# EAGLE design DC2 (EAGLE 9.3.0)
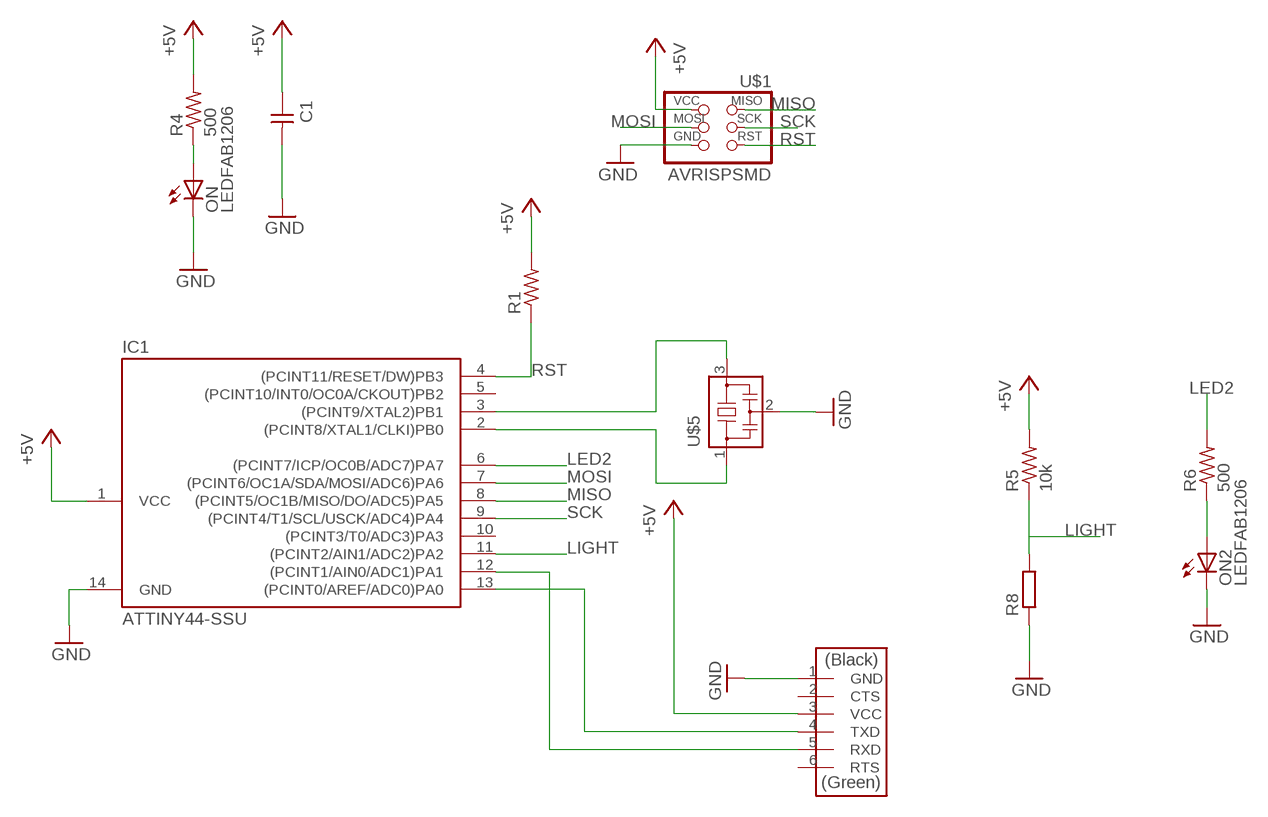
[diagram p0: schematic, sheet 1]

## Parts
C1  CAP-UNPOLARIZEDFAB  [C1206FAB]
IC1  ATTINY44-SSU  [SOIC14]
ON  LEDFAB1206  [LED1206FAB]
ON2  LEDFAB1206  [LED1206FAB]
R1  RES-US1206FAB  [R1206FAB]
R4  500  RES-US1206FAB  [R1206FAB]
R5  10k  RES-US1206FAB  [R1206FAB]
R6  500  RES-US1206FAB  [R1206FAB]
R8  R-EU_0207/10  [0207/10]
U$1  AVRISPSMD  [2X03SMD]
U$2  FTDI-SMD-HEADER  [1X06SMD]
U$5  RESONATOR  [EFOBM]

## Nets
+5V: C1.1 IC1.1(VCC) R1.2 R4.2 R5.2 U$1.2(VCC) U$2.3(VCC)
GND: C1.2 IC1.14(GND) ON2.2(C) ON.2(C) R8.1 U$1.6(GND) U$2.1(GND) U$5.2
LED2: IC1.6((PCINT7/ICP/OC0B/ADC7)PA7) R6.2
LIGHT: IC1.11((PCINT2/AIN1/ADC2)PA2) R5.1 R8.2
MISO: IC1.8((PCINT5/OC1B/MISO/DO/ADC5)PA5) U$1.1(MISO)
MOSI: IC1.7((PCINT6/OC1A/SDA/MOSI/ADC6)PA6) U$1.4(MOSI)
N$1: IC1.2((PCINT8/XTAL1/CLKI)PB0) U$5.1
N$3: IC1.13((PCINT0/AREF/ADC0)PA0) U$2.4(TXD)
N$4: IC1.12((PCINT1/AIN0/ADC1)PA1) U$2.5(RXD)
N$5: IC1.3((PCINT9/XTAL2)PB1) U$5.3
N$6: ON2.1(A) R6.1
N$9: ON.1(A) R4.1
RST: IC1.4((PCINT11/RESET/DW)PB3) R1.1 U$1.5(RST)
SCK: IC1.9((PCINT4/T1/SCL/USCK/ADC4)PA4) U$1.3(SCK)
Unconnected: IC1.5((PCINT10/INT0/OC0A/CKOUT)PB2) IC1.10((PCINT3/T0/ADC3)PA3) U$2.2(CTS) U$2.6(RTS)

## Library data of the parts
C1 = fab:CAP-UNPOLARIZED
IC1 = fab:ATTINY44
ON ON2 = fab:LED: LED
R1 R4-R6 = fab:RES-US: Resistor (US Symbol)
R8 = rcl:R-EU_: RESISTOR, European symbol; SPICEPREFIX: R
U$1 = fab:AVRISP
U$2 = fab:FTDI-SMD-HEADER
U$5 = fab:RESONATOR

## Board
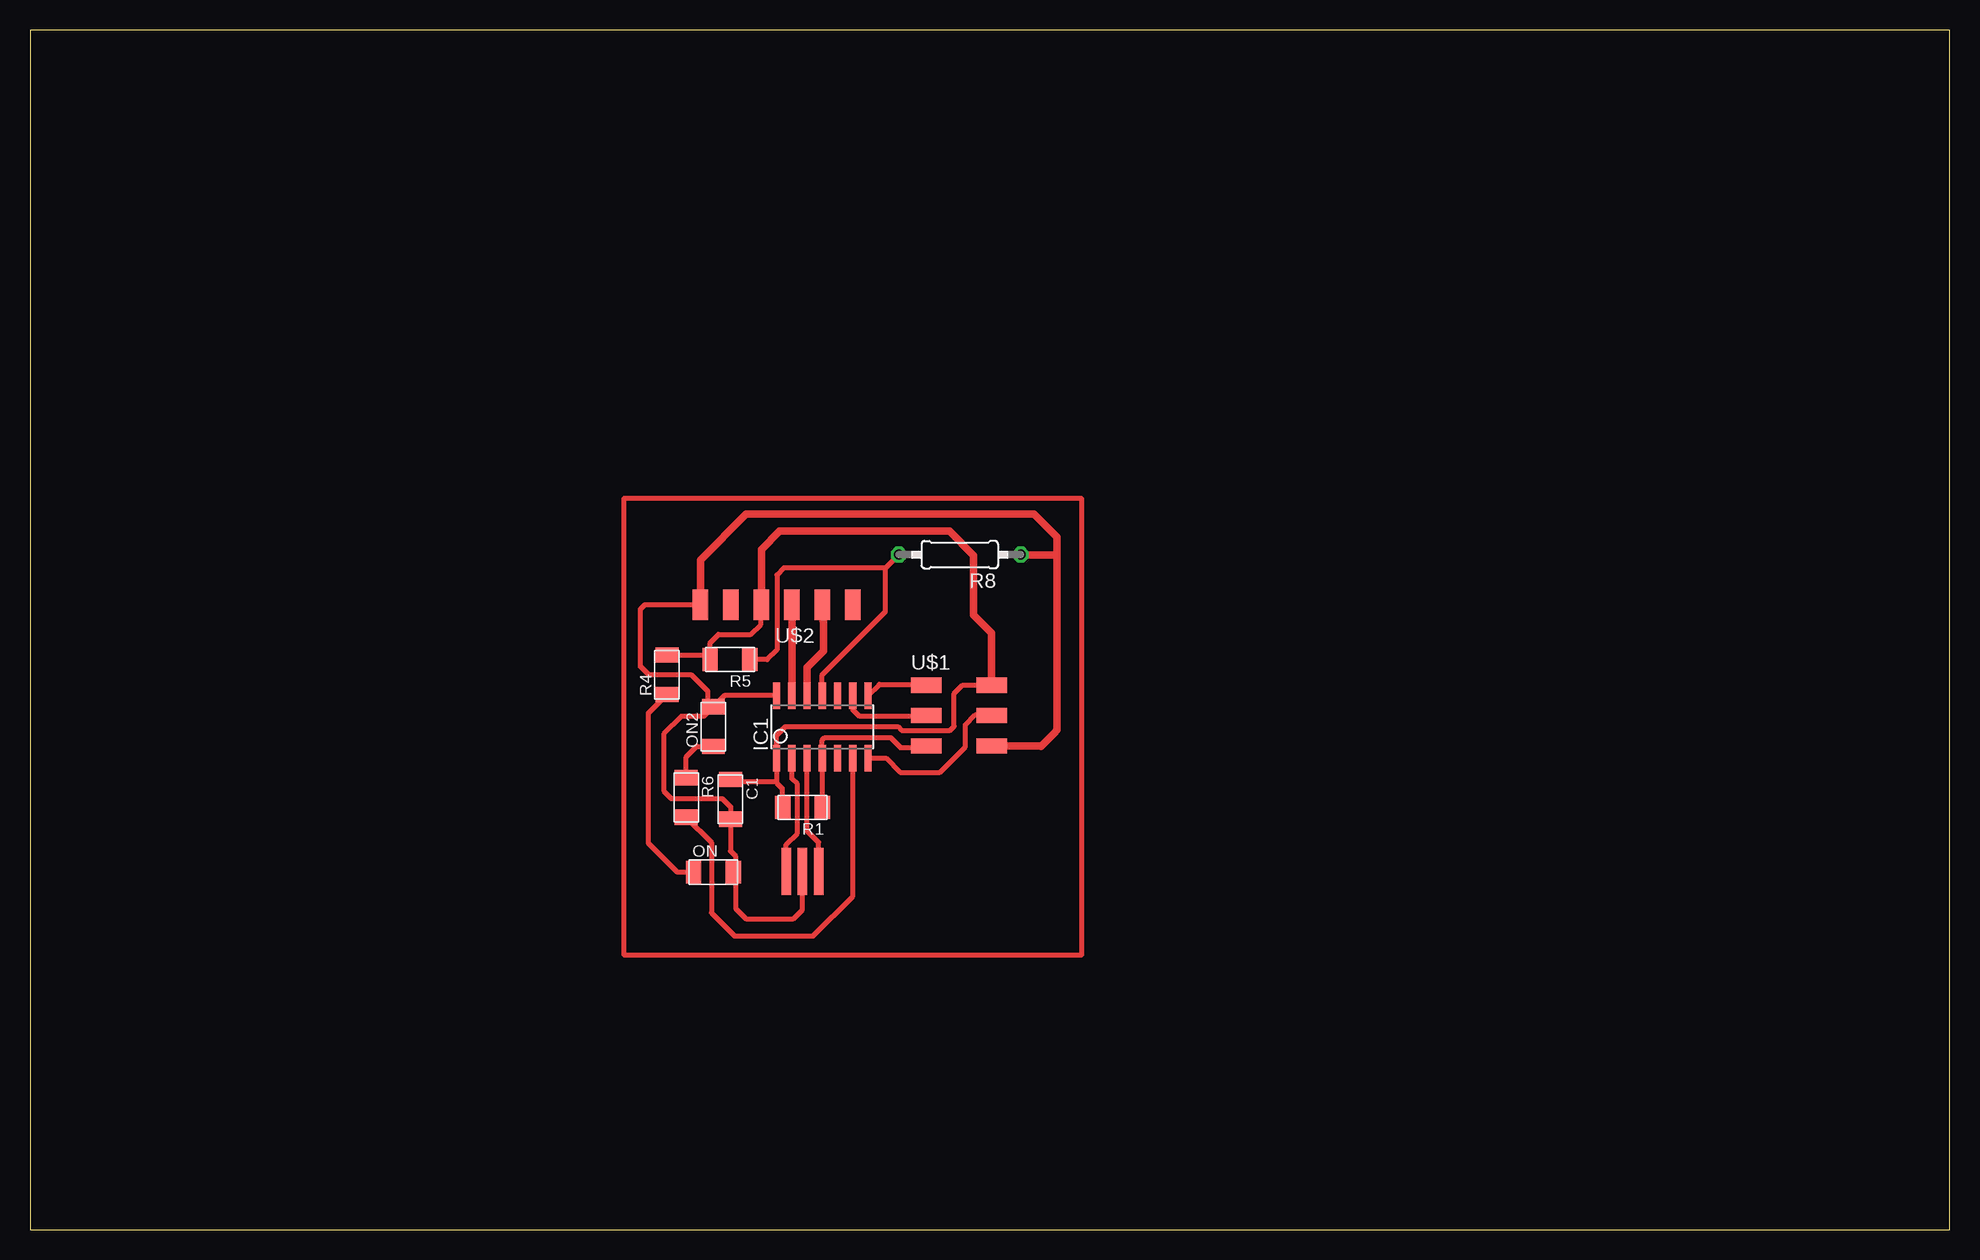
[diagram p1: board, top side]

Size 160 x 100 mm. Coordinates in mm from the lower left corner, seen from the top.
Outline: 0,0 160,0 160,100 0,100 0,0
Copper layers (1*16): Top 0.035mm / dielectric 1.5mm / Bottom 0.035mm
Design rules "default": minimum track width 6mil, minimum drill 0.35mm, track to track 6mil, track to pad 6mil, pad to pad 6mil, via to via 6mil, smd to smd 6mil, copper to edge 40mil, drill to drill 6mil, minimum pad ring 10mil, minimum via ring 8mil, stop-mask expansion 4mil, vias tented up to drill 0mil, thermal gap 10mil

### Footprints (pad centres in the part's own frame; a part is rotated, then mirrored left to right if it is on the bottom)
C1206FAB = smd 1.27 x 1.905: 1 -1.651,0; 2 1.651,0
SOIC14 = smd 0.61 x 2.21: 1 -3.81,-2.603; 2 -2.54,-2.603; 3 -1.27,-2.603; 4 0,-2.603; 5 1.27,-2.603; 6 2.54,-2.603; 7 3.81,-2.603; 8 3.81,2.603; 9 2.54,2.603; 10 1.27,2.603; 11 0,2.603; 12 -1.27,2.603; 13 -2.54,2.603; 14 -3.81,2.603
LED1206FAB = smd 1.27 x 1.905: 1 -1.651,0; 2 1.651,0
R1206FAB = smd 1.27 x 1.905: 1 -1.651,0; 2 1.651,0
0207/10 = drill 0.813 octagon: 1 -5.08,0; 2 5.08,0
2X03SMD = smd 2.54 x 1.27: 1 -2.54,2.54; 2 2.92,2.54; 3 -2.54,0; 4 2.92,0; 5 -2.54,-2.54; 6 2.92,-2.54
1X06SMD = smd 2.54 x 1.27: 1 0,6.35; 2 0,3.81; 3 0,1.27; 4 0,-1.27; 5 0,-3.81; 6 0,-6.35
EFOBM = smd 0.8 x 3.9: 1 -1.35,0; 2 0,0; 3 1.35,0

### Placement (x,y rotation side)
C1  58.39,35.87 270 top
IC1  66.04,41.91 0 top
ON  56.97,29.79 0 top
ON2  56.95,41.92 90 top
R1  64.4,35.19 180 top
R4  53.09,46.25 90 top
R5  58.35,47.52 180 top
R6  54.7,36.02 270 top
R8  77.5,56.26 180 top
U$1  77.24,42.84 0 top
U$2  62.23,52.07 90 top
U$5  64.39,29.86 0 top

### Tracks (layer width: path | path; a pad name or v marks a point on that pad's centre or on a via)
+5V
  Top 0.152: U$1.2 80.16,46.26
  Top 0.406: U$2.3 60.93,52.1 | U$1.2 80.21,45.43 80.64,45.43 80.6,45.39 77.75,45.39 77.04,44.68 77.04,41.95 76.7,41.6 72.66,41.6 72.35,41.92 62.97,41.92 62.23,41.19 IC1.1 62.23,37.35 | 62.23,37.35 62.23,37.25 62.7,36.78 62.7,35.23 R1.2 | 56.7,47.78 56.7,48.91 57.4,49.61 60.08,49.61 60.93,50.46 60.93,52.1 | 60.93,52.1 60.87,52.16 | R4.2 56.58,47.9 56.7,47.78 | 56.7,46.97 R5.2 56.7,47.78 | C1.1 58.56,37.35 62.23,37.35
  Top 0.61: U$1.2 80.16,49.72 78.67,51.22 78.67,56.19 76.63,58.22 62.48,58.22 60.96,56.7 U$2.3
GND
  Top 0.406: 55.83,52.12 U$2.1 51.23,52.07 50.86,51.7 50.86,46.96 51.6,46.21 55.15,46.21 56.51,44.86 56.51,44.02 ON2.2 | U$1.6 | ON.2 58.81,29.6 | U$5.2 64.39,26.66 63.64,25.91 59.68,25.91 58.83,26.76 58.83,29.57 58.81,29.6 | 56.95,43.74 ON2.2 | 58.81,29.6 58.81,31.13 58.39,31.55 C1.2 58.39,35.22 58.4,35.23 57.7,35.93 53.45,35.93 52.82,36.57 52.82,41.3 54.29,42.77 56.15,42.77 ON2.2 | IC1.14 57.89,44.51 ON2.2 | 82.58,55.81 R8.1
  Top 0.61: R8.1 82.61,56.23 85.61,56.23 | U$1.6 84.22,40.3 84.25,40.27 85.34,41.35 85.61,41.62 85.61,56.23 | 85.61,56.23 85.6,56.25 85.6,57.74 83.68,59.65 59.7,59.65 55.88,55.83 U$2.1
LED2
  Top 0.406: R6.2 56.8,32.27 56.8,26.4 58.73,24.48 65.29,24.48 68.6,27.79 68.6,39.29 IC1.6
LIGHT
  Top 0.406: IC1.11 66.04,46.24 71.31,51.51 71.31,55.15 | 71.31,55.15 R8.2 | 71.31,55.15 62.83,55.15 62.25,54.57 62.25,48.32 61.45,47.52 R5.1
MISO
  Top 0.406: 74.64,45.45 U$1.1 74.63,45.46 70.8,45.46 IC1.8 69.92,44.51
MOSI
  Top 0.406: U$1.4 80.12,42.89 78.78,42.89 77.97,42.08 77.97,40.24 75.84,38.12 72.54,38.12 71.35,39.31 IC1.7
N$1
  Top 0.406: U$5.1 63.04,32.09 63.97,33.03 63.97,37.13 63.52,37.58 63.52,38.6 | 63.52,38.6 63.6,38.68 | 63.52,38.6 63.52,39.29 IC1.2
N$2
  Top 0.406: 49.53,60.96 87.63,60.96 87.63,22.86 49.53,22.86 49.53,60.96
N$3
  Top 0.406: 63.5,50.13 U$2.4
  Top 0.61: IC1.13 63.5,50.13 63.5,51.27 63.54,51.3
N$4
  Top 0.406: 66.16,50.51 66.04,50.63 U$2.5
  Top 0.61: IC1.12 64.77,46.85 66.16,48.24 66.16,50.51 66.16,51.04 66.06,51.14
N$5
  Top 0.406: U$5.3 65.74,32.28 64.77,33.24 IC1.3
N$6
  Top 0.406: R6.1 54.7,39.39 55.58,40.27 ON2.1
N$9
  Top 0.406: ON.1 53.96,29.79 51.55,32.21 51.55,43.06 R4.1
RST
  Top 0.406: U$1.5 74.58,40.18 72.55,40.18 72.55,40.2 71.74,41.01 66.25,41.01 66.04,40.81 IC1.4 R1.1
SCK
  Top 0.406: IC1.9 68.57,44.5 68.57,43.35 69.09,42.83 74.04,42.83 74.26,42.61 74.5,42.84 U$1.3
